|   IBIS model for TI xxx DSP
[IBIS Ver]   5.1
[Disclaimer]   Please be aware that in the absence of a written agreement
|   Texas Instruments(TI) assumes no liability for:
|   (1) The accuracy of the IBIS models provided to your company,
|   however, the IBIS model is compliant to industry standard
|   IQ Level 2a.  Refer to IBIS Quality Section below for
|   for full details.
|   (2) The proper functioning of these Models in your design
|   or for any resulting applications
|   (3) Infringement of patents, copyrights or intellectual
|   property rights resulting from your use of these
|   models.
|   TI provides IBIS Models as a service to our customers and
|   therefore reserves the right to limit distribution of the
|   Models.  The information is subject to change without notice.
[File Name]  sprm789.ibs
[File Rev]   0.1
|   -Initial version
|   -Updated Package model
[Date]   18 Oct 2021
[Source]   Texas Instruments Incorporated
[Copyright]   Property of Texas Instruments Incorporated.
|   Unauthorized reproduction and/or distribution is strictly.
|   prohibited.
|   This product is protected under copyright law and trade
|   secret law as an unpublished work.
|   Created 2012,(C) Copyright 1999-2012,
|   Texas Instruments Incorporated., All Rights Reserved.
|   These commodities are under the U.S. Government
|   distribution license control. As such,they are not to be
|   re-exported without the prior approval of the U.S.
|   Department of Commerce.
[Notes]
   ADC pins are marked as NC
   Clock pins are marked as NC
   nReset pin marked as NC
|   Revision History
|   GERNERAL COMMENT: All IBIS Quality Notes below reflect latest release
|   and version of IBIS File
|   File passes ibischk6.0 with 0 errors and 125 warnings
|   Component AM273
[Component] AM273
[Manufacturer] Texas Instruments
[Package Model] AM273_pkg
[Package]
|   typ   min   max
R_pkg   0.20891   0.13735   0.27236
L_pkg   3.388e-9   1.867e-9   4.755e-9
C_pkg   4.07e-13   2.704e-13   6.13e-13
[Pin] Signal_name model_name | Buffer Name
R2	ADC1   NC
P2	ADC2   NC
R1	ADC3   NC
P1	ADC4   NC
M2	ADC5   NC
T2	ADC6   NC
N2	ADC7   NC
N1	ADC8   NC
M1	ADC9   NC
U1	CLKM   NC
V1	CLKP   NC
B6	CSI2_RX0CLKM		CAMERARX_CORE
A6	CSI2_RX0CLKP		CAMERARX_CORE
A8	CSI2_RX0M0		CAMERARX_ADDON
A7	CSI2_RX0M1		CAMERARX_ADDON
B5	CSI2_RX0M2		CAMERARX_ADDON
B4	CSI2_RX0M3		CAMERARX_ADDON
B8	CSI2_RX0P0		CAMERARX_ADDON
B7	CSI2_RX0P1		CAMERARX_ADDON
A5	CSI2_RX0P2		CAMERARX_ADDON
A4	CSI2_RX0P3		CAMERARX_ADDON
A11	CSI2_RX1CLKM		CAMERARX_CORE
B11	CSI2_RX1CLKP		CAMERARX_CORE
A13	CSI2_RX1M0		CAMERARX_ADDON
B12	CSI2_RX1M1		CAMERARX_ADDON
A10	CSI2_RX1M2		CAMERARX_ADDON
A9	CSI2_RX1M3		CAMERARX_ADDON
B13	CSI2_RX1P0		CAMERARX_ADDON
A12	CSI2_RX1P1		CAMERARX_ADDON
B10	CSI2_RX1P2		CAMERARX_ADDON
B9	CSI2_RX1P3		CAMERARX_ADDON
H19	DSS_UARTA_RX		bc1833dv40dcpbfbp18ll_ssdlv
J19	DSS_UARTA_TX		bc1833dv40dcpbfbp18ll_ssdlv
H1	FE1_REFCLK		bc1833dv40dcpbfbp18ll_ssdlv
J2	FE2_REFCLK		bc1833dv40dcpbfbp18ll_ssdlv
V17	HW_SYNC_FE1		bc1833dv40dcpbfbp18ll_ssdlh
W17	HW_SYNC_FE2		bc1833dv40dcpbfbp18ll_ssdlh
W7	LVDS_CLKM		olvds18_ssdhh
V7	LVDS_CLKP		olvds18_ssdhh
W8	LVDS_FRCLKM		olvds18_ssdhh
V8	LVDS_FRCLKP		olvds18_ssdhh
V6	LVDS_TXM0		olvds18_ssdhh
V5	LVDS_TXM1		olvds18_ssdhh
V4	LVDS_TXM2		olvds18_ssdhh
V3	LVDS_TXM3		olvds18_ssdhh
W6	LVDS_TXP0		olvds18_ssdhh
W5	LVDS_TXP1		olvds18_ssdhh
W4	LVDS_TXP2		olvds18_ssdhh
W3	LVDS_TXP3		olvds18_ssdhh
E3	MSS_EPWMA0		bc1833dv40dcpbfbp18ll_ssdlv
B18	MSS_GPIO_10		bc1833dv40dcpbfbp18ll_ssdlh
C17	MSS_GPIO_11		bc1833dv40dcpbfbp18ll_ssdlh
A18	MSS_GPIO_12		bc1833dv40dcpbfbp18ll_ssdlh
B17	MSS_GPIO_13		bc1833dv40dcpbfbp18ll_ssdlh
H2	MSS_GPIO_2		bc1833dv40dcpbfbp18ll_ssdlv
G3	MSS_GPIO_28		bc1833dv40dcpbfbp18ll_ssdlv
B3	MSS_GPIO_8		bc1833dv40dcpbfbp18ll_ssdlv
B19	MSS_GPIO_9		bc1833dv40dcpbfbp18ll_ssdlh
F18	MSS_I2CA_SCL		bc1833dv40dcpbfbp18ll_ssdlv
F16	MSS_I2CA_SDA		bc1833dv40dcpbfbp18ll_ssdlv
B2	MSS_MCANA_RX		bc1833dv40dcpbfbp18ll_ssdlv
A2	MSS_MCANA_TX		bc1833dv40dcpbfbp18ll_ssdlv
C1	MSS_MCANB_RX		bc1833dv40dcpbfbp18ll_ssdlv
B1	MSS_MCANB_TX		bc1833dv40dcpbfbp18ll_ssdlv
R19	MSS_MDIO_CLK		bc1833dv40dcpbfbp18ll_ssdlv
P19	MSS_MDIO_DATA		bc1833dv40dcpbfbp18ll_ssdlv
G19	MSS_MIBSPIA_CLK		bc1833dv40dcpbfbp18ll_ssdlv
F19	MSS_MIBSPIA_CS0		bc1833dv40dcpbfbp18ll_ssdlv
G18	MSS_MIBSPIA_HOSTIRQ	bc1833dv40dcpbfbp18ll_ssdlv
G17	MSS_MIBSPIA_MISO	bc1833dv40dcpbfbp18ll_ssdlv
H18	MSS_MIBSPIA_MOSI	bc1833dv40dcpbfbp18ll_ssdlv
D18	MSS_MIBSPIB_CLK		bc1833dv40dcpbfbp18ll_ssdlv
D19	MSS_MIBSPIB_CS0		bc1833dv40dcpbfbp18ll_ssdlv
E18	MSS_MIBSPIB_CS1		bc1833dv40dcpbfbp18ll_ssdlv
E17	MSS_MIBSPIB_CS2		bc1833dv40dcpbfbp18ll_ssdlv
C19	MSS_MIBSPIB_MISO	bc1833dv40dcpbfbp18ll_ssdlv
C18	MSS_MIBSPIB_MOSI	bc1833dv40dcpbfbp18ll_ssdlv
C2	MSS_QSPI_0		bc1833dv40dcpbfbp18ll_ssdlv
D2	MSS_QSPI_1		bc1833dv40dcpbfbp18ll_ssdlv
D1	MSS_QSPI_2		bc1833dv40dcpbfbp18ll_ssdlv
E2	MSS_QSPI_3		bc1833dv40dcpbfbp18ll_ssdlv
E1	MSS_QSPI_CLK		bc1833dv40dcpbfbp18ll_ssdlv
F2	MSS_QSPI_CS		bc1833dv40dcpbfbp18ll_ssdlv
M19	MSS_RGMII_RCLK		bc1833dv40dcpbfbp18ll_ssdlv
J17	MSS_RGMII_RCTL		bc1833dv40dcpbfbp18ll_ssdlv
P18	MSS_RGMII_RD0		bc1833dv40dcpbfbp18ll_ssdlv
N19	MSS_RGMII_RD1		bc1833dv40dcpbfbp18ll_ssdlv
M18	MSS_RGMII_RD2		bc1833dv40dcpbfbp18ll_ssdlv
L19	MSS_RGMII_RD3		bc1833dv40dcpbfbp18ll_ssdlv
K19	MSS_RGMII_TCLK		bc1833dv40dcpbfbp18ll_ssdlv
J18	MSS_RGMII_TCTL		bc1833dv40dcpbfbp18ll_ssdlv
L18	MSS_RGMII_TD0		bc1833dv40dcpbfbp18ll_ssdlv
L17	MSS_RGMII_TD1		bc1833dv40dcpbfbp18ll_ssdlv
K16	MSS_RGMII_TD2		bc1833dv40dcpbfbp18ll_ssdlv
K18	MSS_RGMII_TD3		bc1833dv40dcpbfbp18ll_ssdlv
G2	MSS_RS232_RX		bc1833dv40dcpbfbp18ll_ssdlv
G1	MSS_RS232_TX		bc1833dv40dcpbfbp18ll_ssdlv
U3	MSS_UARTA_RX		bc1833dv40dcpbfbp18ll_ssdlh
W2	MSS_UARTA_TX		bc1833dv40dcpbfbp18ll_ssdlh
V9	MSS_UARTB_TX		bc1833dv40dcpbfbp18ll_ssdlh
L3	nERROR_IN		bc1833dv40dcpbfbp18ll_od_fs_ssdlv
L1	nERROR_OUT		bc1833dv40dcpbfbp18ll_od_fs_ssdlv
C15	NERRORIN_FE1		bc1833dv40dcpbfbp18ll_ssdlh
A16	NERRORIN_FE2		bc1833dv40dcpbfbp18ll_ssdlh
L2	NRESET   NC
B15	NRESET_FE1		bc1833dv40dcpbfbp18ll_ssdlh
A15	NRESET_FE2		bc1833dv40dcpbfbp18ll_ssdlh
B14	NWARMRESET_IN_FE1	bc1833dv40dcpbfbp18ll_ssdlh
C13	NWARMRESET_IN_FE2	bc1833dv40dcpbfbp18ll_ssdlh
T4	OSC_CLK_OUT_AUDIO	NC
F1	PMIC_CLKOUT		bc1833dv40dcpbfbp18ll_ssdlv
E19	RCSS_GPIO_49		bc1833dv40dcpbfbp18ll_ssdlv
T18	RCSS_MIBSPIA_CLK	bc1833dv40dcpbfbp18ll_ssdlv
T19	RCSS_MIBSPIA_CS0	bc1833dv40dcpbfbp18ll_ssdlv
U18	RCSS_MIBSPIA_HOSTIRQ	bc1833dv40dcpbfbp18ll_ssdlv
R17	RCSS_MIBSPIA_MISO	bc1833dv40dcpbfbp18ll_ssdlv
R18	RCSS_MIBSPIA_MOSI	bc1833dv40dcpbfbp18ll_ssdlv
V19	RCSS_MIBSPIB_CLK	bc1833dv40dcpbfbp18ll_ssdlv
U17	RCSS_MIBSPIB_CS0	bc1833dv40dcpbfbp18ll_ssdlh
W18	RCSS_MIBSPIB_HOSTIRQ	bc1833dv40dcpbfbp18ll_ssdlh
V18	RCSS_MIBSPIB_MISO	bc1833dv40dcpbfbp18ll_ssdlv
U19	RCSS_MIBSPIB_MOSI	bc1833dv40dcpbfbp18ll_ssdlv
B16	RCSS_UARTA_RX		bc1833dv40dcpbfbp18ll_ssdlh
A17	RCSS_UARTA_TX		bc1833dv40dcpbfbp18ll_ssdlh
C3	TCK   bc1833dv40dcpbfbp18ll_ssdlh
C5	TDI   bc1833dv40dcpbfbp18ll_ssdlh
D6	TDO   bc1833dv40dcpbfbp18ll_ssdlh
P4	Temp_Sensor_1		NC
N3	Temp_Sensor_2		NC
D4	TMS   bc1833dv40dcpbfbp18ll_ssdlh
W12	TRACE_CLK		bc1833dv40dcpbfbp18ll_ssdlh
V12	TRACE_CTL		bc1833dv40dcpbfbp18ll_ssdlh
V16	TRACE_DATA_0		bc1833dv40dcpbfbp18ll_ssdlh
U15	TRACE_DATA_1		bc1833dv40dcpbfbp18ll_ssdlh
U11	TRACE_DATA_10		bc1833dv40dcpbfbp18ll_ssdlh
V11	TRACE_DATA_11		bc1833dv40dcpbfbp18ll_ssdlh
W11	TRACE_DATA_12		bc1833dv40dcpbfbp18ll_ssdlh
V10	TRACE_DATA_13		bc1833dv40dcpbfbp18ll_ssdlh
W10	TRACE_DATA_14		bc1833dv40dcpbfbp18ll_ssdlh
T10	TRACE_DATA_15		bc1833dv40dcpbfbp18ll_ssdlh
W16	TRACE_DATA_2		bc1833dv40dcpbfbp18ll_ssdlh
V15	TRACE_DATA_3		bc1833dv40dcpbfbp18ll_ssdlh
W15	TRACE_DATA_4		bc1833dv40dcpbfbp18ll_ssdlh
V14	TRACE_DATA_5		bc1833dv40dcpbfbp18ll_ssdlh
U13	TRACE_DATA_6		bc1833dv40dcpbfbp18ll_ssdlh
W14	TRACE_DATA_7		bc1833dv40dcpbfbp18ll_ssdlh
V13	TRACE_DATA_8		bc1833dv40dcpbfbp18ll_ssdlh
W13	TRACE_DATA_9		bc1833dv40dcpbfbp18ll_ssdlh
T1	VBGAP   NC
E11	VDD   POWER
E9	VDD   POWER
F11	VDD   POWER
F9	VDD   POWER
G14	VDD   POWER
G15	VDD   POWER
G5	VDD   POWER
G6	VDD   POWER
J14	VDD   POWER
J15	VDD   POWER
J5	VDD   POWER
J6	VDD   POWER
L14	VDD   POWER
L15	VDD   POWER
L5	VDD   POWER
L6	VDD   POWER
N14	VDD   POWER
N15	VDD   POWER
N5	VDD   POWER
N6	VDD   POWER
P11	VDD   POWER
P9	VDD   POWER
R11	VDD   POWER
R9	VDD   POWER
N17	VDD_SRAM1		POWER
J3	VDD_SRAM2		POWER
T8	VDD_SRAM3		POWER
D14	VIOIN   POWER
F4	VIOIN   POWER
H16	VIOIN   POWER
K4	VIOIN   POWER
P16	VIOIN   POWER
R5	VIOIN   POWER
T12	VIOIN   POWER
E15	VIOIN_18		POWER
H4	VIOIN_18		POWER
M16	VIOIN_18		POWER
M4	VIOIN_18		POWER
T14	VIOIN_18		POWER
R3	VIOIN_18ADC		POWER
U2	VIOIN_18CLK		POWER
C11	VIOIN_18CSI		POWER
C9	VIOIN_18CSI		POWER
U5	VIOIN_18LVDS		POWER
U7	VIOIN_18LVDS		POWER
N18	VNWA   POWER
U9	VPP   POWER
A1	VSS   GND
A14	VSS   GND
A19	VSS   GND
A3	VSS   GND
C7	VSS   GND
D10	VSS   GND
D12	VSS   GND
D16	VSS   GND
D8	VSS   GND
E12	VSS   GND
E13	VSS   GND
E5	VSS   GND
E7	VSS   GND
E8	VSS   GND
F12	VSS   GND
F13	VSS   GND
F14	VSS   GND
F6	VSS   GND
F7	VSS   GND
F8	VSS   GND
G10	VSS   GND
G11	VSS   GND
G12	VSS   GND
G13	VSS   GND
G7	VSS   GND
G8	VSS   GND
G9	VSS   GND
H10	VSS   GND
H11	VSS   GND
H12	VSS   GND
H13	VSS   GND
H7	VSS   GND
H8	VSS   GND
H9	VSS   GND
J10	VSS   GND
J11	VSS   GND
J12	VSS   GND
J13	VSS   GND
J7	VSS   GND
J8	VSS   GND
J9	VSS   GND
K10	VSS   GND
K11	VSS   GND
K12	VSS   GND
K13	VSS   GND
K7	VSS   GND
K8	VSS   GND
K9	VSS   GND
L10	VSS   GND
L11	VSS   GND
L12	VSS   GND
L13	VSS   GND
L7	VSS   GND
L8	VSS   GND
L9	VSS   GND
M10	VSS   GND
M11	VSS   GND
M12	VSS   GND
M13	VSS   GND
M7	VSS   GND
M8	VSS   GND
M9	VSS   GND
N10	VSS   GND
N11	VSS   GND
N12	VSS   GND
N13	VSS   GND
N7	VSS   GND
N8	VSS   GND
N9	VSS   GND
P12	VSS   GND
P13	VSS   GND
P14	VSS   GND
P6	VSS   GND
P7	VSS   GND
P8	VSS   GND
R12	VSS   GND
R13	VSS   GND
R15	VSS   GND
R7	VSS   GND
R8	VSS   GND
T16	VSS   GND
T6	VSS   GND
V2	VSS   GND
W1	VSS   GND
W19	VSS   GND
W9	VSS   GND
K1	Warm_Reset		bc1833dv40dcpbfbp18ll_od_fs_ssdlv
J1	XREF_CLK0		bc1833dv40dcpbfbp18ll_ssdlv
K2	XREF_CLK1		bc1833dv40dcpbfbp18ll_ssdlv
|   DIFF PIN
[Diff_pin]   inv_pin vdiff tdelay_typ   tdelay_min  tdelay_max
B6	A6	200mV	NA	NA	NA||	CSI2_RX0CLKM	CSI2_RX0CLKP
A8	B8	200mV	NA	NA	NA||	CSI2_RX0M0	CSI2_RX0P0
A7	B7	200mV	NA	NA	NA||	CSI2_RX0M1	CSI2_RX0P1
B5	A5	200mV	NA	NA	NA||	CSI2_RX0M2	CSI2_RX0P2
B4	A4	200mV	NA	NA	NA||	CSI2_RX0M3	CSI2_RX0P3
A11	B11	200mV	NA	NA	NA||	CSI2_RX1CLKM	CSI2_RX1CLKP
A13	B13	200mV	NA	NA	NA||	CSI2_RX1M0	CSI2_RX1P0
B12	A12	200mV	NA	NA	NA||	CSI2_RX1M1	CSI2_RX1P1
A10	B10	200mV	NA	NA	NA||	CSI2_RX1M2	CSI2_RX1P2
A9	B9	200mV	NA	NA	NA||	CSI2_RX1M3	CSI2_RX1P3
W7	V7	200mV	NA	NA	NA||	LVDS_CLKM	LVDS_CLKP
W8	V8	200mV	NA	NA	NA||	LVDS_FRCLKM	LVDS_FRCLKP
V6	W6	200mV	NA	NA	NA||	LVDS_TXM0	LVDS_TXP0
V5	W5	200mV	NA	NA	NA||	LVDS_TXM1	LVDS_TXP1
V4	W4	200mV	NA	NA	NA||	LVDS_TXM2	LVDS_TXP2
V3	W3	200mV	NA	NA	NA||	LVDS_TXM3	LVDS_TXP3
|   SERIES PIN MAPPING
[Series Pin Mapping] pin_2 model_name function_table_group
 A8	B8	s_CAMERARX_ADDON_HSRX
 A7	B7	s_CAMERARX_ADDON_HSRX
 B5	A5	s_CAMERARX_ADDON_HSRX
 B4	A4   s_CAMERARX_ADDON_HSRX
 A6   B6   s_CAMERARX_CORE_HSRX
 A13	B13	s_CAMERARX_ADDON_HSRX
 A12	B12	s_CAMERARX_ADDON_HSRX
 A10	B10	s_CAMERARX_ADDON_HSRX
 B9	A9   s_CAMERARX_ADDON_HSRX
 A11   B11   s_CAMERARX_CORE_HSRX
|   CAMERARX_ADDON
[Model Selector] CAMERARX_ADDON
CAMERARX_ADDON_PD_ON  Cell operated at 1.8(nom)
|CAMERARX_ADDON_PD_ON_1P8PIPU_0_ON & PIPD_0_OFF
CAMERARX_ADDON_PU_ON  Cell operated at 1.8(nom)
|CAMERARX_ADDON_PU_ON_1P8PIPU_0_OFF & PIPD_0_ON
CAMERARX_ADDON_PUPD0  Cell operated at 1.8(nom)
|CAMERARX_ADDON_PUPD_OFF_1P8PIPU_0_ON & PIPD_0_ON
CAMERARX_ADDON_HSRX  High Speed RX
CAMERARX_ADDON_LPRX  Low Power RX
CAMERARX_ADDON_ULPRX  Ultra Low Power RX
|   CAMERA_RX_CORE
[Model Selector] CAMERARX_CORE
CAMERARX_CORE_PD_ON  Cell operated at 1.8(nom)
|CAMERARX_CORE_PD_ON_1P8PIPU_0_ON & PIPD_0_OFF
CAMERARX_CORE_PU_ON  Cell operated at 1.8(nom)
|CAMERARX_CORE_PU_ON_1P8PIPU_0_OFF & PIPD_0_ON
CAMERARX_CORE_PUPD0  Cell operated at 1.8(nom)
|CAMERARX_CORE_PUPD_OFF_1P8PIPU_0_ON & PIPD_0_ON
CAMERARX_CORE_HSRX  High Speed RX
CAMERARX_CORE_LPRX  Low Power RX
CAMERARX_CORE_ULPRX  Ultra Low Power RX
|   BC1833DV40DCPBFBP18LL_SSDLH
[Model Selector] bc1833dv40dcpbfbp18ll_ssdlh
|SC1 IS A SLEW RATE CONTROL PIN
|5% SUPPLY VARIATION MODES WITH 1.8V NOM SUPPLY
BC40D_H_PUPDOFF_5P_SC1_1P8  Cell operated at 1.8(nom)
|BC40D_H_PUPDOFF_5P_SC1_1P8; BUFFER WITH WEAK PULUP/PULLDOWN OFF AT 5% SUPPLY
|VARIATION WITH SC1=1 MEANING SLOW MODE OF OPERATION
BC40D_H_PD_ON_5P_!SC1_1P8  Cell operated at 1.8(nom)
|BC40D_H_PD_ON_5P_!SC1_1P8; BUFFER WITH WEAK_PULLDOWN_ON AT 5% SUPPLY
|VARIATION WITH SC1=0 MEANING FAST MODE OF OPERATION
BC40D_H_PD_ON_5P_SC1_1P8  Cell operated at 1.8(nom)
|BC40D_H_PD_ON_5P_SC1_1P8; BUFFER WITH WEAK_PULLDOWN_ON AT 5% SUPPLY
|VARIATION WITH SC1=1 MEANING SLOW MODE OF OPERATION
BC40D_H_PU_ON_5P_!SC1_1P8  Cell operated at 1.8(nom)
|BC40D_H_PU_ON_5P_!SC1_1P8; BUFFER WITH WEAK_PULLUP_ON AT 5% SUPPLY
|VARIATION WITH SC1=0 MEANING FAST MODE OF OPERATION
BC40D_H_PUPDOFF_5P_!SC1_1P8  Cell operated at 1.8(nom)
|BC40D_H_PUPDOFF_5P_!SC1_1P8; BUFFER WITH WEAK PULUP/PULLDOWN OFF AT 5% SUPPLY
|VARIATION WITH SC1=0 MEANING FAST MODE OF OPERATION
BC40D_H_PU_ON_5P_SC1_1P8  Cell operated at 1.8(nom)
|BC40D_H_PU_ON_5P_SC1_1P8; BUFFER WITH WEAK_PULLUP_ON AT 5% SUPPLY
|VARIATION WITH SC1=1 MEANING SLOW MODE OF OPERATION
|5% SUPPLY VARIATION MODES WITH 3.3V NOM SUPPLY
BC40D_H_PUPDOFF_5P_SC1_3P3  Cell operated at 3.3(nom)
|BC40D_H_PUPDOFF_5P_SC1_3P3; BUFFER WITH WEAK PULUP/PULLDOWN OFF AT 5% SUPPLY
|VARIATION WITH SC1=1 MEANING SLOW MODE OF OPERATION
BC40D_H_PD_ON_5P_!SC1_3P3  Cell operated at 3.3(nom)
|BC40D_H_PD_ON_5P_!SC1_3P3; BUFFER WITH WEAK_PULLDOWN_ON AT 5% SUPPLY
|VARIATION WITH SC1=0 MEANING FAST MODE OF OPERATION
BC40D_H_PD_ON_5P_SC1_3P3  Cell operated at 3.3(nom)
|BC40D_H_PD_ON_5P_SC1_3P3; BUFFER WITH WEAK_PULLDOWN_ON AT 5% SUPPLY
|VARIATION WITH SC1=1 MEANING SLOW MODE OF OPERATION
BC40D_H_PU_ON_5P_!SC1_3P3  Cell operated at 3.3(nom)
|BC40D_H_PU_ON_5P_!SC1_3P3; BUFFER WITH WEAK_PULLUP_ON AT 5% SUPPLY
|VARIATION WITH SC1=0 MEANING FAST MODE OF OPERATION
BC40D_H_PUPDOFF_5P_!SC1_3P3  Cell operated at 3.3(nom)
|BC40D_H_PUPDOFF_5P_!SC1_3P3; BUFFER WITH WEAK PULUP/PULLDOWN OFF AT 5% SUPPLY
|VARIATION WITH SC1=0 MEANING FAST MODE OF OPERATION
BC40D_H_PU_ON_5P_SC1_3P3  Cell operated at 3.3(nom)
|BC40D_H_PU_ON_5P_SC1_3P3; BUFFER WITH WEAK_PULLUP_ON AT 5% SUPPLY
|VARIATION WITH SC1=1 MEANING SLOW MODE OF OPERATION
| 10% SUPPLY VARIATION MODES WITH 1.8V NOM SUPPLY
BC40D_H_PUPDOFF_10P_SC1_1P8  Cell operated at 1.8(nom)
|BC40D_H_PUPDOFF_10P_SC1_1P8; BUFFER WITH WEAK PULUP/PULLDOWN OFF AT 10% SUPPLY
|VARIATION WITH SC1=1 MEANING SLOW MODE OF OPERATION
BC40D_H_PD_ON_10P_!SC1_1P8  Cell operated at 1.8(nom)
|BC40D_H_PD_ON_10P_!SC1_1P8; BUFFER WITH WEAK_PULLDOWN_ON AT 10% SUPPLY
|VARIATION WITH SC1=0 MEANING FAST MODE OF OPERATION
BC40D_H_PD_ON_10P_SC1_1P8  Cell operated at 1.8(nom)
|BC40D_H_PD_ON_10P_SC1_1P8; BUFFER WITH WEAK_PULLDOWN_ON AT 10% SUPPLY
|VARIATION WITH SC1=1 MEANING SLOW MODE OF OPERATION
BC40D_H_PU_ON_10P_!SC1_1P8  Cell operated at 1.8(nom)
|BC40D_H_PU_ON_10P_!SC1_1P8; BUFFER WITH WEAK_PULLUP_ON AT 10% SUPPLY
|VARIATION WITH SC1=0 MEANING FAST MODE OF OPERATION
BC40D_H_PUPDOFF_10P_!SC1_1P8  Cell operated at 1.8(nom)
|BC40D_H_PUPDOFF_10P_!SC1_1P8; BUFFER WITH WEAK PULUP/PULLDOWN OFF AT 10% SUPPLY
|VARIATION WITH SC1=0 MEANING FAST MODE OF OPERATION
BC40D_H_PU_ON_10P_SC1_1P8  Cell operated at 1.8(nom)
|BC40D_H_PU_ON_10P_SC1_1P8; BUFFER WITH WEAK_PULLUP_ON AT 10% SUPPLY
|VARIATION WITH SC1=1 MEANING SLOW MODE OF OPERATION
| 10% SUPPLY VARIATION MODES WITH 3.3V NOM SUPPLY
BC40D_H_PUPDOFF_10P_SC1_3P3  Cell operated at 3.3(nom)
|BC40D_H_PUPDOFF_10P_SC1_3P3; BUFFER WITH WEAK PULUP/PULLDOWN OFF AT 10% SUPPLY
|VARIATION WITH SC1=1 MEANING SLOW MODE OF OPERATION
BC40D_H_PD_ON_10P_!SC1_3P3  Cell operated at 3.3(nom)
|BC40D_H_PD_ON_10P_!SC1_3P3; BUFFER WITH WEAK_PULLDOWN_ON 10% SUPPLY
|VARIATION WITH SC1=0 MEANING FAST MODE OF OPERATION
BC40D_H_PD_ON_10P_SC1_3P3  Cell operated at 3.3(nom)
|BC40D_H_PD_ON_10P_SC1_3P3; BUFFER WITH WEAK_PULLDOWN_ON AT 10% SUPPLY
|VARIATION WITH SC1=1 MEANING SLOW MODE OF OPERATION
BC40D_H_PU_ON_10P_!SC1_3P3  Cell operated at 3.3(nom)
|BC40D_H_PU_ON_10P_!SC1_3P3; BUFFER WITH WEAK_PULLUP_ON AT 10% SUPPLY
|VARIATION WITH SC1=0 MEANING FAST MODE OF OPERATION
BC40D_H_PUPDOFF_10P_!SC1_3P3  Cell operated at 3.3(nom)
|BC40D_H_PUPDOFF_10P_!SC1_3P3; BUFFER WITH WEAK PULUP/PULLDOWN OFF AT 10% SUPPLY
|VARIATION WITH SC1=0 MEANING FAST MODE OF OPERATION
BC40D_H_PU_ON_10P_SC1_3P3  Cell operated at 3.3(nom)
|BC40D_H_PU_ON_10P_SC1_3P3; BUFFER WITH WEAK_PULLUP_ON AT 10% SUPPLY
|VARIATION WITH SC1=1 MEANING SLOW MODE OF OPERATION
|   BC1833DV40DCPBFBP18LL_SSDLV
[Model Selector] bc1833dv40dcpbfbp18ll_ssdlv
|SC1 IS A SLEW RATE CONTROL PIN
|5% SUPPLY VARIATION MODES WITH 1.8V NOM SUPPLY
BC40D_V_PUPDOFF_5P_SC1_1P8  Cell operated at 1.8(nom)
|BC40D_V_PUPDOFF_5P_SC1_1P8; BUFFER WITH WEAK PULUP/PULLDOWN OFF AT 5% SUPPLY
|VARIATION WITH SC1=1 MEANING SLOW MODE OF OPERATION
BC40D_V_PD_ON_5P_!SC1_1P8  Cell operated at 1.8(nom)
|BC40D_V_PD_ON_5P_!SC1_1P8; BUFFER WITH WEAK_PULLDOWN_ON AT 5% SUPPLY
|VARIATION WITH SC1=0 MEANING FAST MODE OF OPERATION
BC40D_V_PD_ON_5P_SC1_1P8  Cell operated at 1.8(nom)
|BC40D_V_PD_ON_5P_SC1_1P8; BUFFER WITH WEAK_PULLDOWN_ON AT 5% SUPPLY
|VARIATION WITH SC1=1 MEANING SLOW MODE OF OPERATION
BC40D_V_PU_ON_5P_!SC1_1P8  Cell operated at 1.8(nom)
|BC40D_V_PU_ON_5P_!SC1_1P8; BUFFER WITH WEAK_PULLUP_ON AT 5% SUPPLY
|VARIATION WITH SC1=0 MEANING FAST MODE OF OPERATION
BC40D_V_PUPDOFF_5P_!SC1_1P8  Cell operated at 1.8(nom)
|BC40D_V_PUPDOFF_5P_!SC1_1P8; BUFFER WITH WEAK PULUP/PULLDOWN OFF AT 5% SUPPLY
|VARIATION WITH SC1=0 MEANING FAST MODE OF OPERATION
BC40D_V_PU_ON_5P_SC1_1P8  Cell operated at 1.8(nom)
|BC40D_V_PU_ON_5P_SC1_1P8; BUFFER WITH WEAK_PULLUP_ON AT 5% SUPPLY
|VARIATION WITH SC1=1 MEANING SLOW MODE OF OPERATION
|5% SUPPLY VARIATION MODES WITH 3.3V NOM SUPPLY
BC40D_V_PUPDOFF_5P_SC1_3P3  Cell operated at 3.3(nom)
|BC40D_V_PUPDOFF_5P_SC1_3P3; BUFFER WITH WEAK PULUP/PULLDOWN OFF AT 5% SUPPLY
|VARIATION WITH SC1=1 MEANING SLOW MODE OF OPERATION
BC40D_V_PD_ON_5P_!SC1_3P3  Cell operated at 3.3(nom)
|BC40D_V_PD_ON_5P_!SC1_3P3; BUFFER WITH WEAK_PULLDOWN_ON AT 5% SUPPLY
|VARIATION WITH SC1=0 MEANING FAST MODE OF OPERATION
BC40D_V_PD_ON_5P_SC1_3P3  Cell operated at 3.3(nom)
|BC40D_V_PD_ON_5P_SC1_3P3; BUFFER WITH WEAK_PULLDOWN_ON AT 5% SUPPLY
|VARIATION WITH SC1=1 MEANING SLOW MODE OF OPERATION
BC40D_V_PU_ON_5P_!SC1_3P3  Cell operated at 3.3(nom)
|BC40D_V_PU_ON_5P_!SC1_3P3; BUFFER WITH WEAK_PULLUP_ON AT 5% SUPPLY
|VARIATION WITH SC1=0 MEANING FAST MODE OF OPERATION
BC40D_V_PUPDOFF_5P_!SC1_3P3  Cell operated at 3.3(nom)
|BC40D_V_PUPDOFF_5P_!SC1_3P3; BUFFER WITH WEAK PULUP/PULLDOWN OFF AT 5% SUPPLY
|VARIATION WITH SC1=0 MEANING FAST MODE OF OPERATION
BC40D_V_PU_ON_5P_SC1_3P3  Cell operated at 3.3(nom)
|BC40D_V_PU_ON_5P_SC1_3P3; BUFFER WITH WEAK_PULLUP_ON AT 5% SUPPLY
|VARIATION WITH SC1=1 MEANING SLOW MODE OF OPERATION
| 10% SUPPLY VARIATION MODES WITH 1.8V NOM SUPPLY
BC40D_V_PUPDOFF_10P_SC1_1P8  Cell operated at 1.8(nom)
|BC40D_V_PUPDOFF_10P_SC1_1P8; BUFFER WITH WEAK PULUP/PULLDOWN OFF AT 10% SUPPLY
|VARIATION WITH SC1=1 MEANING SLOW MODE OF OPERATION
BC40D_V_PD_ON_10P_!SC1_1P8  Cell operated at 1.8(nom)
|BC40D_V_PD_ON_10P_!SC1_1P8; BUFFER WITH WEAK_PULLDOWN_ON AT 10% SUPPLY
|VARIATION WITH SC1=0 MEANING FAST MODE OF OPERATION
BC40D_V_PD_ON_10P_SC1_1P8  Cell operated at 1.8(nom)
|BC40D_V_PD_ON_10P_SC1_1P8; BUFFER WITH WEAK_PULLDOWN_ON AT 10% SUPPLY
|VARIATION WITH SC1=1 MEANING SLOW MODE OF OPERATION
BC40D_V_PU_ON_10P_!SC1_1P8  Cell operated at 1.8(nom)
|BC40D_V_PU_ON_10P_!SC1_1P8; BUFFER WITH WEAK_PULLUP_ON AT 10% SUPPLY
|VARIATION WITH SC1=0 MEANING FAST MODE OF OPERATION
BC40D_V_PUPDOFF_10P_!SC1_1P8  Cell operated at 1.8(nom)
|BC40D_V_PUPDOFF_10P_!SC1_1P8; BUFFER WITH WEAK PULUP/PULLDOWN OFF AT 10% SUPPLY
|VARIATION WITH SC1=0 MEANING FAST MODE OF OPERATION
BC40D_V_PU_ON_10P_SC1_1P8  Cell operated at 1.8(nom)
|BC40D_V_PU_ON_10P_SC1_1P8; BUFFER WITH WEAK_PULLUP_ON AT 10% SUPPLY
|VARIATION WITH SC1=1 MEANING SLOW MODE OF OPERATION
| 10% SUPPLY VARIATION MODES WITH 3.3V NOM SUPPLY
BC40D_V_PUPDOFF_10P_SC1_3P3  Cell operated at 3.3(nom)
|BC40D_V_PUPDOFF_10P_SC1_3P3; BUFFER WITH WEAK PULUP/PULLDOWN OFF AT 10% SUPPLY
|VARIATION WITH SC1=1 MEANING SLOW MODE OF OPERATION
BC40D_V_PD_ON_10P_!SC1_3P3  Cell operated at 3.3(nom)
|BC40D_V_PD_ON_10P_!SC1_3P3; BUFFER WITH WEAK_PULLDOWN_ON 10% SUPPLY
|VARIATION WITH SC1=0 MEANING FAST MODE OF OPERATION
BC40D_V_PD_ON_10P_SC1_3P3  Cell operated at 3.3(nom)
|BC40D_V_PD_ON_10P_SC1_3P3; BUFFER WITH WEAK_PULLDOWN_ON AT 10% SUPPLY
|VARIATION WITH SC1=1 MEANING SLOW MODE OF OPERATION
BC40D_V_PU_ON_10P_!SC1_3P3  Cell operated at 3.3(nom)
|BC40D_V_PU_ON_10P_!SC1_3P3; BUFFER WITH WEAK_PULLUP_ON AT 10% SUPPLY
|VARIATION WITH SC1=0 MEANING FAST MODE OF OPERATION
BC40D_V_PUPDOFF_10P_!SC1_3P3  Cell operated at 3.3(nom)
|BC40D_V_PUPDOFF_10P_!SC1_3P3; BUFFER WITH WEAK PULUP/PULLDOWN OFF AT 10% SUPPLY
|VARIATION WITH SC1=0 MEANING FAST MODE OF OPERATION
BC40D_V_PU_ON_10P_SC1_3P3  Cell operated at 3.3(nom)
|BC40D_V_PU_ON_10P_SC1_3P3; BUFFER WITH WEAK_PULLUP_ON AT 10% SUPPLY
|VARIATION WITH SC1=1 MEANING SLOW MODE OF OPERATION
|   BC1833DV40DCPBFBP18LL_OD_FS_SSDLV
[Model Selector] bc1833dv40dcpbfbp18ll_od_fs_ssdlv
|SC1 IS A SLEW RATE CONTROL PIN
|5% SUPPLY VARIATION MODES WITH 1.8V NOM SUPPLY
BC40D_V_PUPDOFF_5P_SC1_1P8  Cell operated at 1.8(nom)
|BC40D_V_PUPDOFF_5P_SC1_1P8; BUFFER WITH WEAK PULUP/PULLDOWN OFF AT 5% SUPPLY
|VARIATION WITH SC1=1 MEANING SLOW MODE OF OPERATION
BC40D_V_PD_ON_5P_!SC1_1P8  Cell operated at 1.8(nom)
|BC40D_V_PD_ON_5P_!SC1_1P8; BUFFER WITH WEAK_PULLDOWN_ON AT 5% SUPPLY
|VARIATION WITH SC1=0 MEANING FAST MODE OF OPERATION
BC40D_V_PD_ON_5P_SC1_1P8  Cell operated at 1.8(nom)
|BC40D_V_PD_ON_5P_SC1_1P8; BUFFER WITH WEAK_PULLDOWN_ON AT 5% SUPPLY
|VARIATION WITH SC1=1 MEANING SLOW MODE OF OPERATION
BC40D_V_PU_ON_5P_!SC1_1P8  Cell operated at 1.8(nom)
|BC40D_V_PU_ON_5P_!SC1_1P8; BUFFER WITH WEAK_PULLUP_ON AT 5% SUPPLY
|VARIATION WITH SC1=0 MEANING FAST MODE OF OPERATION
BC40D_V_PUPDOFF_5P_!SC1_1P8  Cell operated at 1.8(nom)
|BC40D_V_PUPDOFF_5P_!SC1_1P8; BUFFER WITH WEAK PULUP/PULLDOWN OFF AT 5% SUPPLY
|VARIATION WITH SC1=0 MEANING FAST MODE OF OPERATION
BC40D_V_PU_ON_5P_SC1_1P8  Cell operated at 1.8(nom)
|BC40D_V_PU_ON_5P_SC1_1P8; BUFFER WITH WEAK_PULLUP_ON AT 5% SUPPLY
|VARIATION WITH SC1=1 MEANING SLOW MODE OF OPERATION
|5% SUPPLY VARIATION MODES WITH 3.3V NOM SUPPLY
BC40D_V_PUPDOFF_5P_SC1_3P3  Cell operated at 3.3(nom)
|BC40D_V_PUPDOFF_5P_SC1_3P3; BUFFER WITH WEAK PULUP/PULLDOWN OFF AT 5% SUPPLY
|VARIATION WITH SC1=1 MEANING SLOW MODE OF OPERATION
BC40D_V_PD_ON_5P_!SC1_3P3  Cell operated at 3.3(nom)
|BC40D_V_PD_ON_5P_!SC1_3P3; BUFFER WITH WEAK_PULLDOWN_ON AT 5% SUPPLY
|VARIATION WITH SC1=0 MEANING FAST MODE OF OPERATION
BC40D_V_PD_ON_5P_SC1_3P3  Cell operated at 3.3(nom)
|BC40D_V_PD_ON_5P_SC1_3P3; BUFFER WITH WEAK_PULLDOWN_ON AT 5% SUPPLY
|VARIATION WITH SC1=1 MEANING SLOW MODE OF OPERATION
BC40D_V_PU_ON_5P_!SC1_3P3  Cell operated at 3.3(nom)
|BC40D_V_PU_ON_5P_!SC1_3P3; BUFFER WITH WEAK_PULLUP_ON AT 5% SUPPLY
|VARIATION WITH SC1=0 MEANING FAST MODE OF OPERATION
BC40D_V_PUPDOFF_5P_!SC1_3P3  Cell operated at 3.3(nom)
|BC40D_V_PUPDOFF_5P_!SC1_3P3; BUFFER WITH WEAK PULUP/PULLDOWN OFF AT 5% SUPPLY
|VARIATION WITH SC1=0 MEANING FAST MODE OF OPERATION
BC40D_V_PU_ON_5P_SC1_3P3  Cell operated at 3.3(nom)
|BC40D_V_PU_ON_5P_SC1_3P3; BUFFER WITH WEAK_PULLUP_ON AT 5% SUPPLY
|VARIATION WITH SC1=1 MEANING SLOW MODE OF OPERATION
| 10% SUPPLY VARIATION MODES WITH 1.8V NOM SUPPLY
BC40D_V_PUPDOFF_10P_SC1_1P8  Cell operated at 1.8(nom)
|BC40D_V_PUPDOFF_10P_SC1_1P8; BUFFER WITH WEAK PULUP/PULLDOWN OFF AT 10% SUPPLY
|VARIATION WITH SC1=1 MEANING SLOW MODE OF OPERATION
BC40D_V_PD_ON_10P_!SC1_1P8  Cell operated at 1.8(nom)
|BC40D_V_PD_ON_10P_!SC1_1P8; BUFFER WITH WEAK_PULLDOWN_ON AT 10% SUPPLY
|VARIATION WITH SC1=0 MEANING FAST MODE OF OPERATION
BC40D_V_PD_ON_10P_SC1_1P8  Cell operated at 1.8(nom)
|BC40D_V_PD_ON_10P_SC1_1P8; BUFFER WITH WEAK_PULLDOWN_ON AT 10% SUPPLY
|VARIATION WITH SC1=1 MEANING SLOW MODE OF OPERATION
BC40D_V_PU_ON_10P_!SC1_1P8  Cell operated at 1.8(nom)
|BC40D_V_PU_ON_10P_!SC1_1P8; BUFFER WITH WEAK_PULLUP_ON AT 10% SUPPLY
|VARIATION WITH SC1=0 MEANING FAST MODE OF OPERATION
BC40D_V_PUPDOFF_10P_!SC1_1P8  Cell operated at 1.8(nom)
|BC40D_V_PUPDOFF_10P_!SC1_1P8; BUFFER WITH WEAK PULUP/PULLDOWN OFF AT 10% SUPPLY
|VARIATION WITH SC1=0 MEANING FAST MODE OF OPERATION
BC40D_V_PU_ON_10P_SC1_1P8  Cell operated at 1.8(nom)
|BC40D_V_PU_ON_10P_SC1_1P8; BUFFER WITH WEAK_PULLUP_ON AT 10% SUPPLY
|VARIATION WITH SC1=1 MEANING SLOW MODE OF OPERATION
| 10% SUPPLY VARIATION MODES WITH 3.3V NOM SUPPLY
BC40D_V_PUPDOFF_10P_SC1_3P3  Cell operated at 3.3(nom)
|BC40D_V_PUPDOFF_10P_SC1_3P3; BUFFER WITH WEAK PULUP/PULLDOWN OFF AT 10% SUPPLY
|VARIATION WITH SC1=1 MEANING SLOW MODE OF OPERATION
BC40D_V_PD_ON_10P_!SC1_3P3  Cell operated at 3.3(nom)
|BC40D_V_PD_ON_10P_!SC1_3P3; BUFFER WITH WEAK_PULLDOWN_ON 10% SUPPLY
|VARIATION WITH SC1=0 MEANING FAST MODE OF OPERATION
BC40D_V_PD_ON_10P_SC1_3P3  Cell operated at 3.3(nom)
|BC40D_V_PD_ON_10P_SC1_3P3; BUFFER WITH WEAK_PULLDOWN_ON AT 10% SUPPLY
|VARIATION WITH SC1=1 MEANING SLOW MODE OF OPERATION
BC40D_V_PU_ON_10P_!SC1_3P3  Cell operated at 3.3(nom)
|BC40D_V_PU_ON_10P_!SC1_3P3; BUFFER WITH WEAK_PULLUP_ON AT 10% SUPPLY
|VARIATION WITH SC1=0 MEANING FAST MODE OF OPERATION
BC40D_V_PUPDOFF_10P_!SC1_3P3  Cell operated at 3.3(nom)
|BC40D_V_PUPDOFF_10P_!SC1_3P3; BUFFER WITH WEAK PULUP/PULLDOWN OFF AT 10% SUPPLY
|VARIATION WITH SC1=0 MEANING FAST MODE OF OPERATION
BC40D_V_PU_ON_10P_SC1_3P3  Cell operated at 3.3(nom)
|BC40D_V_PU_ON_10P_SC1_3P3; BUFFER WITH WEAK_PULLUP_ON AT 10% SUPPLY
|VARIATION WITH SC1=1 MEANING SLOW MODE OF OPERATION
|   OLVDS
[Model Selector] olvds18_ssdhh
OLVDS18_SSDHH_4MA_100_SUBLVDS_1P8  Cell operated at 1.8(nom)
|OLVDS18_SSDHH_4MA_100_SUBLVDS_1P8; SUB_LVDS 4MA OUTPUT CURRENT SETTING WIT
|H 100 OHM INTERNAL TERMINATION
OLVDS18_SSDHH_2.5MA_100_LVDS_1P8  Cell operated at 1.8(nom)
|OLVDS18_SSDHH_2.5MA_100_LVDS_1P8; LVDS 2.5MA OUTPUT CURRENT SETTING WITH 1
|00 OHM INTERNAL TERMINATION
OLVDS18_SSDHH_3MA_100_LVDS_1P8  Cell operated at 1.8(nom)
|OLVDS18_SSDHH_3MA_100_LVDS_1P8; LVDS 3MA OUTPUT CURRENT SETTING WITH 100 O
|HM INTERNAL TERMINATION
OLVDS18_SSDHH_3.33MA_200_LVDS_1P8  Cell operated at 1.8(nom)
|OLVDS18_SSDHH_3.33MA_200_LVDS_1P8; LVDS 3.33MA OUTPUT CURRENT SETTING WITH
| 200 OHM INTERNAL TERMINATION
OLVDS18_SSDHH_2.5MA_100_SUBLVDS_1P8  Cell operated at 1.8(nom)
|OLVDS18_SSDHH_2.5MA_100_SUBLVDS_1P8; SUB_LVDS 2.5MA OUTPUT CURRENT SETTING
| WITH 100 OHM INTERNAL TERMINATION
OLVDS18_SSDHH_4MA_200_LVDS_1P8  Cell operated at 1.8(nom)
|OLVDS18_SSDHH_4MA_200_LVDS_1P8; LVDS 4MA OUTPUT CURRENT SETTING WITH 200 O
|HM INTERNAL TERMINATION
OLVDS18_SSDHH_3MA_100_SUBLVDS_1P8  Cell operated at 1.8(nom)
|OLVDS18_SSDHH_3MA_100_SUBLVDS_1P8; SUB_LVDS 3MA OUTPUT CURRENT SETTING WIT
|H 100 OHM INTERNAL TERMINATION
OLVDS18_SSDHH_3.33MA_200_SUBLVDS_1P8  Cell operated at 1.8(nom)
|OLVDS18_SSDHH_3.33MA_200_SUBLVDS_1P8; SUB_LVDS 3.33MA OUTPUT CURRENT SETTI
|NG WITH 200 OHM INTERNAL TERMINATION
OLVDS18_SSDHH_2MA_200_LVDS_1P8  Cell operated at 1.8(nom)
|OLVDS18_SSDHH_2MA_200_LVDS_1P8; LVDS 2MA OUTPUT CURRENT SETTING WITH 200 O
|HM INTERNAL TERMINATION
OLVDS18_SSDHH_4MA_200_SUBLVDS_1P8  Cell operated at 1.8(nom)
|OLVDS18_SSDHH_4MA_200_SUBLVDS_1P8; SUB_LVDS 4MA OUTPUT CURRENT SETTING WIT
|H 200 OHM INTERNAL TERMINATION
OLVDS18_SSDHH_2.66MA_200_LVDS_1P8  Cell operated at 1.8(nom)
|OLVDS18_SSDHH_2.66MA_200_LVDS_1P8; LVDS 2.66MA OUTPUT CURRENT SETTING WITH
| 200 OHM INTERNAL TERMINATION
OLVDS18_SSDHH_2MA_200_SUBLVDS_1P8  Cell operated at 1.8(nom)
|OLVDS18_SSDHH_2MA_200_SUBLVDS_1P8; SUB_LVDS 2MA OUTPUT CURRENT SETTING WIT
|H 200 OHM INTERNAL TERMINATION
OLVDS18_SSDHH_3.5MA_100_LVDS_1P8  Cell operated at 1.8(nom)
|OLVDS18_SSDHH_3.5MA_100_LVDS_1P8; LVDS 3.5MA OUTPUT CURRENT SETTING WITH 1
|00 OHM INTERNAL TERMINATION
OLVDS18_SSDHH_2.66MA_200_SUBLVDS_1P8  Cell operated at 1.8(nom)
|OLVDS18_SSDHH_2.66MA_200_SUBLVDS_1P8; SUB_LVDS 2.66MA OUTPUT CURRENT SETTI
|NG WITH 200 OHM INTERNAL TERMINATION
OLVDS18_SSDHH_4MA_100_LVDS_1P8  Cell operated at 1.8(nom)
|OLVDS18_SSDHH_4MA_100_LVDS_1P8; LVDS 4MA OUTPUT CURRENT SETTING WITH 100 O
|HM INTERNAL TERMINATION
OLVDS18_SSDHH_3.5MA_100_SUBLVDS_1P8  Cell operated at 1.8(nom)
|   Package Model
[Define Package Model]   AM273_pkg
[Manufacturer]   name 1
[OEM]   name 2
[Description]   164-pin Package
|[Number of Sections]   1
[Number of Pins]   164
[Pin Numbers]
|[Pin Name]  Net Number   Net Name   Net's All Pins
T1   | 1   VBGAP   T1
N6   | 2   VDD   N6
   |N5
   |L6
   |L5
   |J6
   |J5
   |G6
   |G5
   |F9
   |E9
   |P9
   |R9
   |F11
   |E11
   |P11
   |R11
   |G14
   |J14
   |L14
   |N14
   |G15
   |J15
   |L15
   |N15
N17   | 3   VDD_SRAM1   N17
J3   | 4   VDD_SRAM2   J3
T8   | 5   VDD_SRAM3   T8
F4   | 6   VIOIN   F4
   |K4
   |R5
   |T12
   |D14
   |H16
   |P16
H4   | 7   VIOIN_18   H4
   |M4
   |T14
   |E15
   |M16
R3   | 8   VIOIN_18ADC   R3
U2   | 9   VIOIN_18CLK   U2
C11   | 10   VIOIN_18CSI   C11
   |C9
U7   | 11   VIOIN_18LVDS   U7
   |U5
N18   | 12   VNWA   N18
U9   | 13   VPP   U9
R2   | 14   ADC1   R2
P2   | 15   ADC2   P2
R1   | 16   ADC3   R1
P1   | 17   ADC4   P1
M2   | 18   ADC5   M2
T2   | 19   ADC6   T2
N2   | 20   ADC7   N2
N1   | 21   ADC8   N1
M1   | 22   ADC9   M1
U1   | 23   CLKM   U1
V1   | 24   CLKP   V1
B6   | 25   CSI2_RX0CLKM   B6
A6   | 26   CSI2_RX0CLKP   A6
A8   | 27   CSI2_RX0M0   A8
A7   | 28   CSI2_RX0M1   A7
B5   | 29   CSI2_RX0M2   B5
B4   | 30   CSI2_RX0M3   B4
B8   | 31   CSI2_RX0P0   B8
B7   | 32   CSI2_RX0P1   B7
A5   | 33   CSI2_RX0P2   A5
A4   | 34   CSI2_RX0P3   A4
A11   | 35   CSI2_RX1CLKM   A11
B11   | 36   CSI2_RX1CLKP   B11
A13   | 37   CSI2_RX1M0   A13
B12   | 38   CSI2_RX1M1   B12
A10   | 39   CSI2_RX1M2   A10
A9   | 40   CSI2_RX1M3   A9
B13   | 41   CSI2_RX1P0   B13
A12   | 42   CSI2_RX1P1   A12
B10   | 43   CSI2_RX1P2   B10
B9   | 44   CSI2_RX1P3   B9
H19   | 45   DSS_UARTA_RX   H19
J19   | 46   DSS_UARTA_TX   J19
H1   | 47   FE1_REFCLK   H1
J2   | 48   FE2_REFCLK   J2
V17   | 49   HW_SYNC_FE1   V17
W17   | 50   HW_SYNC_FE2   W17
W7   | 51   LVDS_CLKM   W7
V7   | 52   LVDS_CLKP   V7
W8   | 53   LVDS_FRCLKM   W8
V8   | 54   LVDS_FRCLKP   V8
V6   | 55   LVDS_TXM0   V6
V5   | 56   LVDS_TXM1   V5
V4   | 57   LVDS_TXM2   V4
V3   | 58   LVDS_TXM3   V3
W6   | 59   LVDS_TXP0   W6
W5   | 60   LVDS_TXP1   W5
W4   | 61   LVDS_TXP2   W4
W3   | 62   LVDS_TXP3   W3
E3   | 63   MSS_EPWMA0   E3
H2   | 64   MSS_GPIO_2   H2
B3   | 65   MSS_GPIO_8   B3
B19   | 66   MSS_GPIO_9   B19
B18   | 67   MSS_GPIO_10   B18
C17   | 68   MSS_GPIO_11   C17
A18   | 69   MSS_GPIO_12   A18
B17   | 70   MSS_GPIO_13   B17
G3   | 71   MSS_GPIO_28   G3
F18   | 72   MSS_I2CA_SCL   F18
F16   | 73   MSS_I2CA_SDA   F16
B2   | 74   MSS_MCANA_RX   B2
A2   | 75   MSS_MCANA_TX   A2
C1   | 76   MSS_MCANB_RX   C1
B1   | 77   MSS_MCANB_TX   B1
R19   | 78   MSS_MDIO_CLK   R19
P19   | 79   MSS_MDIO_DATA   P19
G19   | 80   MSS_MIBSPIA_CLK   G19
F19   | 81   MSS_MIBSPIA_CS0   F19
G18   | 82   MSS_MIBSPIA_HOSTIRQ   G18
G17   | 83   MSS_MIBSPIA_MISO   G17
H18   | 84   MSS_MIBSPIA_MOSI   H18
D18   | 85   MSS_MIBSPIB_CLK   D18
D19   | 86   MSS_MIBSPIB_CS0   D19
E18   | 87   MSS_MIBSPIB_CS1   E18
E17   | 88   MSS_MIBSPIB_CS2   E17
C19   | 89   MSS_MIBSPIB_MISO   C19
C18   | 90   MSS_MIBSPIB_MOSI   C18
C2   | 91   MSS_QSPI_0   C2
D2   | 92   MSS_QSPI_1   D2
D1   | 93   MSS_QSPI_2   D1
E2   | 94   MSS_QSPI_3   E2
E1   | 95   MSS_QSPI_CLK   E1
F2   | 96   MSS_QSPI_CS   F2
M19   | 97   MSS_RGMII_RCLK   M19
J17   | 98   MSS_RGMII_RCTL   J17
P18   | 99   MSS_RGMII_RD0   P18
N19   | 100   MSS_RGMII_RD1   N19
M18   | 101   MSS_RGMII_RD2   M18
L19   | 102   MSS_RGMII_RD3   L19
K19   | 103   MSS_RGMII_TCLK   K19
J18   | 104   MSS_RGMII_TCTL   J18
L18   | 105   MSS_RGMII_TD0   L18
L17   | 106   MSS_RGMII_TD1   L17
K16   | 107   MSS_RGMII_TD2   K16
K18   | 108   MSS_RGMII_TD3   K18
G2   | 109   MSS_RS232_RX   G2
G1   | 110   MSS_RS232_TX   G1
U3   | 111   MSS_UARTA_RX   U3
W2   | 112   MSS_UARTA_TX   W2
V9   | 113   MSS_UARTB_TX   V9
C15   | 114   NERRORIN_FE1   C15
A16   | 115   NERRORIN_FE2   A16
L3   | 116   NERROR_IN   L3
L1   | 117   NERROR_OUT   L1
L2   | 118   NRESET   L2
B15   | 119   NRESET_FE1   B15
A15   | 120   NRESET_FE2   A15
B14   | 121   NWARMRESET_IN_FE1   B14
C13   | 122   NWARMRESET_IN_FE2   C13
T4   | 123   OSC_CLK_OUT_AUDIO   T4
F1   | 124   PMIC_CLKOUT   F1
E19   | 125   RCSS_GPIO_49   E19
T18   | 126   RCSS_MIBSPIA_CLK   T18
T19   | 127   RCSS_MIBSPIA_CS0   T19
U18   | 128   RCSS_MIBSPIA_HOSTIRQ   U18
R17   | 129   RCSS_MIBSPIA_MISO   R17
R18   | 130   RCSS_MIBSPIA_MOSI   R18
V19   | 131   RCSS_MIBSPIB_CLK   V19
U17   | 132   RCSS_MIBSPIB_CS0   U17
W18   | 133   RCSS_MIBSPIB_HOSTIRQ   W18
V18   | 134   RCSS_MIBSPIB_MISO   V18
U19   | 135   RCSS_MIBSPIB_MOSI   U19
B16   | 136   RCSS_UARTA_RX   B16
A17   | 137   RCSS_UARTA_TX   A17
C3   | 138   TCK   C3
C5   | 139   TDI   C5
D6   | 140   TDO   D6
P4   | 141   TEMP_SENSOR_1   P4
N3   | 142   TEMP_SENSOR_2   N3
D4   | 143   TMS   D4
W12   | 144   TRACE_CLK   W12
V12   | 145   TRACE_CTL   V12
V16   | 146   TRACE_DATA_0   V16
U15   | 147   TRACE_DATA_1   U15
W16   | 148   TRACE_DATA_2   W16
V15   | 149   TRACE_DATA_3   V15
W15   | 150   TRACE_DATA_4   W15
V14   | 151   TRACE_DATA_5   V14
U13   | 152   TRACE_DATA_6   U13
W14   | 153   TRACE_DATA_7   W14
V13   | 154   TRACE_DATA_8   V13
W13   | 155   TRACE_DATA_9   W13
U11   | 156   TRACE_DATA_10   U11
V11   | 157   TRACE_DATA_11   V11
W11   | 158   TRACE_DATA_12   W11
V10   | 159   TRACE_DATA_13   V10
W10   | 160   TRACE_DATA_14   W10
T10   | 161   TRACE_DATA_15   T10
K1   | 162   WARM_RESET   K1
J1   | 163   XREF_CLK0   J1
K2   | 164   XREF_CLK1   K2
[Model Data]
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[End Model Data]
[End Package Model]
[Model]   s_CAMERARX_ADDON_HSRX
Model_type   Series
C_comp   4.13955p   3.54298p   4.784869p
[Voltage Range]   1.8 1.62 1.89
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[Model]   s_CAMERARX_CORE_HSRX
Model_type   Series
C_comp   4.13955p   3.54198p   4.784869p
[Voltage Range]   1.8 1.62 1.92
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| Models and submodels in the file (78): CAMERARX_ADDON_HSRX (Input), s_CAMERARX_ADDON_HSRX (Series), CAMERARX_ADDON_LPRX (Input), CAMERARX_ADDON_ULPRX (Input), CAMERARX_ADDON_PD_ON (Input), CAMERARX_ADDON_PU_ON (Input), CAMERARX_ADDON_PUPD0 (Input), CAMERARX_CORE_HSRX (Input), s_CAMERARX_CORE_HSRX (Series), CAMERARX_CORE_LPRX (Input), CAMERARX_CORE_ULPRX (Input), CAMERARX_CORE_PD_ON (Input), CAMERARX_CORE_PU_ON (Input), CAMERARX_CORE_PUPD0 (Input), OLVDS18_SSDHH_4MA_100_SUBLVDS_1P8 (Output), OLVDS18_SSDHH_2.5MA_100_LVDS_1P8 (Output), OLVDS18_SSDHH_3MA_100_LVDS_1P8 (Output), OLVDS18_SSDHH_3.33MA_200_LVDS_1P8 (Output), OLVDS18_SSDHH_2.5MA_100_SUBLVDS_1P8 (Output), OLVDS18_SSDHH_4MA_200_LVDS_1P8 (Output), OLVDS18_SSDHH_3MA_100_SUBLVDS_1P8 (Output), OLVDS18_SSDHH_3.33MA_200_SUBLVDS_1P8 (Output), OLVDS18_SSDHH_2MA_200_LVDS_1P8 (Output), OLVDS18_SSDHH_4MA_200_SUBLVDS_1P8 (Output), OLVDS18_SSDHH_2.66MA_200_LVDS_1P8 (Output), OLVDS18_SSDHH_2MA_200_SUBLVDS_1P8 (Output), OLVDS18_SSDHH_3.5MA_100_LVDS_1P8 (Output), OLVDS18_SSDHH_2.66MA_200_SUBLVDS_1P8 (Output), OLVDS18_SSDHH_4MA_100_LVDS_1P8 (Output), OLVDS18_SSDHH_3.5MA_100_SUBLVDS_1P8 (Output), BC40D_H_PUPDOFF_5P_SC1_1P8 (I/O), BC40D_H_PD_ON_5P_!SC1_1P8 (I/O), BC40D_H_PD_ON_5P_SC1_1P8 (I/O), BC40D_H_PU_ON_5P_!SC1_1P8 (I/O), BC40D_H_PUPDOFF_5P_!SC1_1P8 (I/O), BC40D_H_PU_ON_5P_SC1_1P8 (I/O), BC40D_H_PUPDOFF_5P_SC1_3P3 (I/O), BC40D_H_PD_ON_5P_!SC1_3P3 (I/O), BC40D_H_PD_ON_5P_SC1_3P3 (I/O), BC40D_H_PU_ON_5P_!SC1_3P3 (I/O), BC40D_H_PUPDOFF_5P_!SC1_3P3 (I/O), BC40D_H_PU_ON_5P_SC1_3P3 (I/O), BC40D_H_PUPDOFF_10P_SC1_1P8 (I/O), BC40D_H_PD_ON_10P_!SC1_1P8 (I/O), BC40D_H_PD_ON_10P_SC1_1P8 (I/O), BC40D_H_PU_ON_10P_!SC1_1P8 (I/O), BC40D_H_PUPDOFF_10P_!SC1_1P8 (I/O), BC40D_H_PU_ON_10P_SC1_1P8 (I/O), BC40D_H_PUPDOFF_10P_SC1_3P3 (I/O), BC40D_H_PD_ON_10P_!SC1_3P3 (I/O), BC40D_H_PD_ON_10P_SC1_3P3 (I/O), BC40D_H_PU_ON_10P_!SC1_3P3 (I/O), BC40D_H_PUPDOFF_10P_!SC1_3P3 (I/O), BC40D_H_PU_ON_10P_SC1_3P3 (I/O), BC40D_V_PUPDOFF_5P_SC1_1P8 (I/O), BC40D_V_PD_ON_5P_!SC1_1P8 (I/O), BC40D_V_PD_ON_5P_SC1_1P8 (I/O), BC40D_V_PU_ON_5P_!SC1_1P8 (I/O), BC40D_V_PUPDOFF_5P_!SC1_1P8 (I/O), BC40D_V_PU_ON_5P_SC1_1P8 (I/O), BC40D_V_PUPDOFF_5P_SC1_3P3 (I/O), BC40D_V_PD_ON_5P_!SC1_3P3 (I/O), BC40D_V_PD_ON_5P_SC1_3P3 (I/O), BC40D_V_PU_ON_5P_!SC1_3P3 (I/O), BC40D_V_PUPDOFF_5P_!SC1_3P3 (I/O), BC40D_V_PU_ON_5P_SC1_3P3 (I/O), BC40D_V_PUPDOFF_10P_SC1_1P8 (I/O), BC40D_V_PD_ON_10P_!SC1_1P8 (I/O), BC40D_V_PD_ON_10P_SC1_1P8 (I/O), BC40D_V_PU_ON_10P_!SC1_1P8 (I/O), BC40D_V_PUPDOFF_10P_!SC1_1P8 (I/O), BC40D_V_PU_ON_10P_SC1_1P8 (I/O), BC40D_V_PUPDOFF_10P_SC1_3P3 (I/O), BC40D_V_PD_ON_10P_!SC1_3P3 (I/O), BC40D_V_PD_ON_10P_SC1_3P3 (I/O), BC40D_V_PU_ON_10P_!SC1_3P3 (I/O), BC40D_V_PUPDOFF_10P_!SC1_3P3 (I/O), BC40D_V_PU_ON_10P_SC1_3P3 (I/O)
